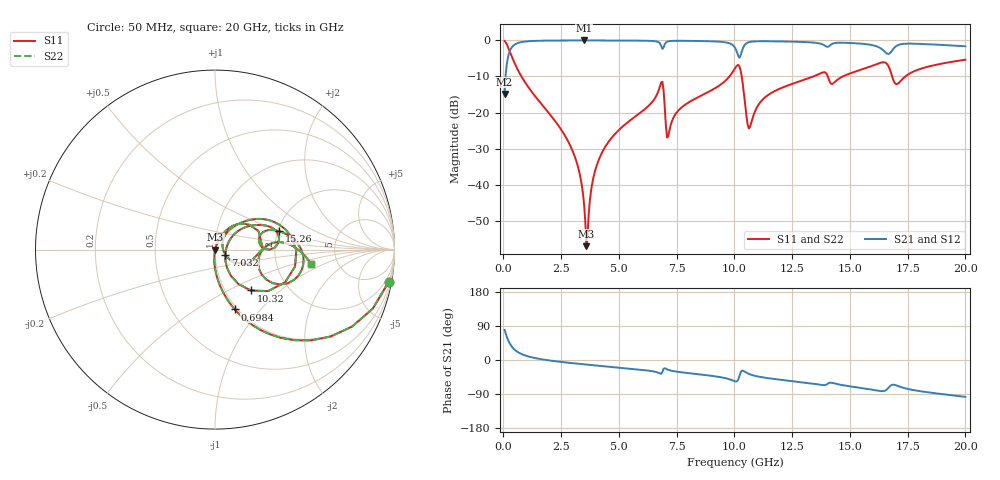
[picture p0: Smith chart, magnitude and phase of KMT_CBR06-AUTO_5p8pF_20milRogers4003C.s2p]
! Data measured by Modelithics Inc. support@modelithics.com 813-866-6335
! KEMET CBR06-AUTO 5.8pF, Pad Width= 0.851mm, Pad Length= 0.64mm, Pad Gap= 0.62mm, 20mil Rogers 4003C substrate Data, January 2022
# hz S ma R 50
! 2 Port Network Data from SP1.SP block
! freq  magS11  angS11  magS21  angS21  magS12  angS12  magS22  angS22
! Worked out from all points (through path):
!   401 points, 50 MHz to 20 GHz, reference 50 ohm
!   highest |S21| = -0.01 dB at 3.491 GHz (marker M1); lowest = -14.9 dB at 50 MHz (marker M2)
!   group delay of S21, straight-line fit = 15.1 ps
!   lowest |S11| = -57.0 dB at 3.591 GHz (marker M3), VSWR 1.00, Z = 50.1 - j0.0934 ohm
!   |S11| at or under -10 dB: 779.8 MHz to 9.783 GHz (9.003 GHz wide, 170 % of centre); 10.31 GHz to 13.42 GHz (3.103 GHz wide, 26.2 % of centre); 14.04 GHz to 14.69 GHz (646.4 MHz wide, 4.5 % of centre)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
!   |S22| runs from -57.0 to -0.1 dB; largest |S21 - S12| = 0
!   S11 on the Smith chart (normalised r, x): 50 MHz: 1, -11; 698.4 MHz: 0.97, -0.74; 7.032 GHz: 1.12, -0.07; 10.32 GHz: 1.31, -0.66; 15.26 GHz: 2.04, +0.48; 20 GHz: 3.18, -0.71
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5e7  0.9835 -10.6  0.1808 79.4  0.1808 79.4  0.9835 -10.6
2.99375e8  0.6699 -48.9  0.7419 41.0  0.7419 41.0  0.6699 -48.9
6.98375e8  0.3515 -71.7  0.9355 18.2  0.9355 18.2  0.3515 -71.7
2.74325e9  0.04316 -95.3  0.9979 -6.8  0.9979 -6.8  0.04316 -95.3
3.391625e9  0.009848 -93.9  0.9986 -10.8  0.9986 -10.8  0.009848 -93.9
3.491375e9  0.005321 -88.3  0.9987 -11.4  0.9987 -11.4  0.005321 -88.3
3.591125e9  0.001406 -41.5  0.9986 -12.0  0.9986 -12.0  0.001406 -41.5
3.94025e9  0.01444 70.8  0.9985 -14.1  0.9985 -14.1  0.01444 70.8
4.289375e9  0.02878 71.2  0.9981 -16.0  0.9981 -16.0  0.02878 71.2
6.73325e9  0.209 44.0  0.9362 -34.3  0.9362 -34.3  0.209 44.0
6.882875e9  0.267 1.2  0.7641 -31.2  0.7641 -31.2  0.267 1.2
7.0325e9  0.0664 -28.6  0.9336 -23.1  0.9336 -23.1  0.0664 -28.6
7.182125e9  0.05568 41.0  0.9775 -26.9  0.9775 -26.9  0.05568 41.0
1.0025e10  0.4106 15.5  0.7914 -56.2  0.7914 -56.2  0.4106 15.5
1.032425e10  0.3029 -48.8  0.7105 -28.1  0.7105 -28.1  0.3029 -48.8
1.067338e10  0.06305 5.9  0.9531 -37.9  0.9531 -37.9  0.06305 5.9
1.14215e10  0.1717 38.7  0.9739 -47.6  0.9739 -47.6  0.1717 38.7
1.336662e10  0.3116 25.5  0.9368 -62.1  0.9368 -62.1  0.3116 25.5
1.526188e10  0.3724 15.8  0.9123 -71.8  0.9123 -71.8  0.3724 15.8
1.670825e10  0.4126 -28.1  0.6558 -70.7  0.6558 -70.7  0.4126 -28.1
1.705738e10  0.2498 -7.5  0.8528 -68.1  0.8528 -68.1  0.2498 -7.5
2e10  0.541 -8.4  0.8298 -97.3  0.8298 -97.3  0.541 -8.4
